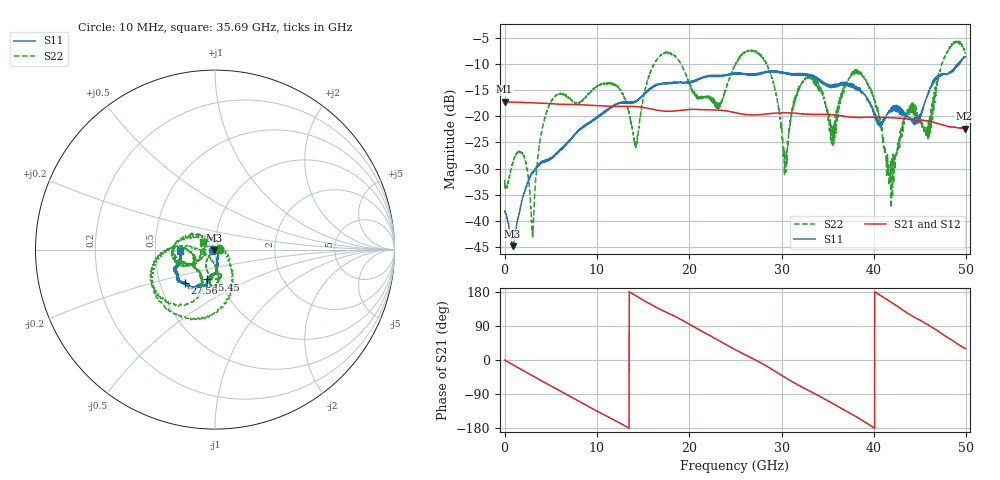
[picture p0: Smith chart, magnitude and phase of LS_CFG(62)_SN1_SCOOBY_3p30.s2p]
!Keysight Technologies,N5245B,MY58422026,A.13.80.08
!Date: Thursday, March 19, 2020 23:46:23
!Correction: S11(Full 2 Port(1,2))
!S21(Full 2 Port(1,2))
!S12(Full 2 Port(1,2))
!S22(Full 2 Port(1,2))
!S2P File: Measurements: S11, S21, S12, S22:
# Hz S DB R 50.0
!freq dBS11 angS11 dBS21 angS21 dBS12 angS12 dBS22 angS22
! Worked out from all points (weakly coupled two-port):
!   4991 points, 10 MHz to 49.91 GHz, reference 50 ohm
!   highest |S21| = -17.24 dB at 10 MHz (marker M1); lowest = -22.4 dB at 49.82 GHz (marker M2)
!   lowest |S11| = -44.8 dB at 870 MHz (marker M3), VSWR 1.01, Z = 49.6 - j0.4 ohm
!   |S11| at or under -10 dB: start of sweep to 49.12 GHz; 49.16824 GHz to 49.22385 GHz (55.61 MHz wide, 0.113 % of centre)
!   |S22| runs from -43.3 to -5.5 dB; largest |S21 - S12| = 0.0014
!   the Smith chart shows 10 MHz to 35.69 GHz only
!   S11 on the Smith chart (normalised r, x): 10 MHz: 0.98, -0.01; 15.45 GHz: 0.87, -0.30; 27.56 GHz: 0.67, -0.27; 35.69 GHz: 0.67, -0.01
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1e7  -38.13 -167.2  -17.24 -0.3  -17.23 -0.3  -32.17 1.6
8.7e8  -44.81 -135.5  -17.30 -12.1  -17.30 -12.1  -29.01 -36.8
2.13e9  -34.63 -56.4  -17.37 -29.4  -17.37 -29.3  -27.62 -12.2
3.03e9  -30.88 -57.1  -17.43 -41.6  -17.43 -41.6  -42.72 -71.6
4.78e9  -28.13 -64.2  -17.58 -65.5  -17.58 -65.4  -18.18 -111.6
8.33e9  -22.42 -80.5  -17.82 -112.7  -17.81 -112.6  -17.14 -91.7
1.208e10  -17.72 -87.9  -18.11 -161.1  -18.11 -161.1  -14.03 -87.6
1.42e10  -17.22 -95.8  -18.15 170.0  -18.14 170.1  -25.58 -132.7
1.545e10  -15.31 -104.3  -18.47 151.9  -18.46 152.0  -13.22 175.5
1.665e10  -13.96 -103.4  -18.88 136.2  -18.87 136.3  -8.85 -164.0
2.312e10  -12.41 -118.2  -18.83 52.4  -18.83 52.6  -18.67 -158.9
2.496e10  -11.91 -123.6  -19.29 27.3  -19.28 27.5  -10.36 -173.1
2.756e10  -11.92 -132.1  -19.71 -4.9  -19.71 -4.7  -8.23 -103.8
3.039e10  -11.75 -144.3  -19.35 -46.2  -19.36 -46.0  -28.49 45.0
3.328e10  -12.27 -156.9  -19.63 -85.2  -19.63 -84.8  -12.58 -166.2
3.569e10  -14.08 -178.1  -19.77 -116.8  -19.71 -116.3  -21.92 150.1
3.85e10  -14.88 175.3  -20.24 -155.7  -20.21 -155.9  -11.81 -156.0
4.16e10  -19.03 105.7  -20.26 156.6  -20.28 156.5  -29.58 92.3
4.675e10  -12.45 7.4  -21.32 79.4  -21.34 79.6  -13.95 -138.5
4.841e10  -11.48 -5.7  -22.09 53.2  -22.12 53.2  -6.26 -64.9
4.982e10  -8.71 -15.1  -22.39 31.0  -22.40 31.2  -7.25 -12.5
4.991e10  -8.64 -14.2  -22.38 30.0  -22.41 30.0  -7.87 -12.8
